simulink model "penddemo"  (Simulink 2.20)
settings: Solver=ode45  StartTime=0  StopTime=10000  MaxStep=0.02  RelTol=1e-3  AbsTol=1e-6

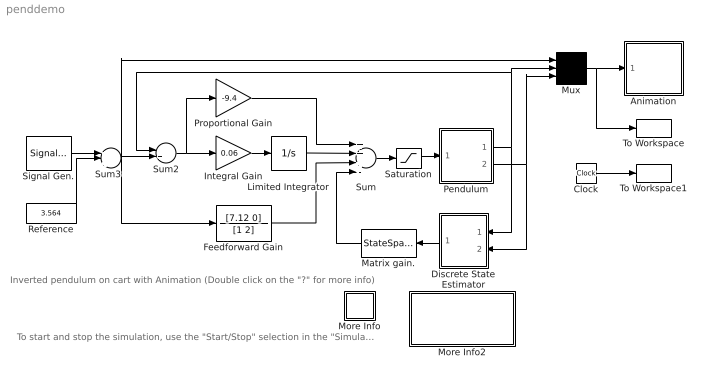
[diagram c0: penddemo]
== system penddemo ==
  note: Inverted pendulum on cart with Animation (Double click on the "?" for more info)
  note: To start and stop the simulation, use the "Start/Stop" selection in the "Simulation" pull-down menu
  Animation : Subsystem  mask(Pendulum plot){}
      mask help: Pendulum plot
      mask init:
      | RefBlock=&1;
  Clock : Clock
  Discrete State Estimator : Subsystem  Orientation=left  mask(Pendulum Discrete state estimator){}
      mask help: Pendulum discrete state estimator
      mask init:
      | Ts = @1;
  Feedforward Gain : TransferFcn  Numerator=[7.12 0]  Denominator=[1 2]
  Integral Gain : Gain  Gain=0.06
  Limited Integrator : Integrator  ExternalReset=none  InitialConditionSource=internal  InitialCondition=0  LimitOutput=on  UpperSaturationLimit=5  LowerSaturationLimit=-5  ShowSaturationPort=off  ShowStatePort=off  AbsoluteTolerance=auto
  Matrix gain. : StateSpace  Orientation=left  A=[]  B=[]  C=[]  D=K  X0=0  mask(Matrix gain){}
      mask help: Matrix Gain:
      mask init:
      | K = @1;
  More Info : Subsystem
  More Info2 : Subsystem
  Mux : Mux  Inputs=3
  Pendulum : Subsystem  mask(Inverted pendulum on cart){}
      mask help: Unmask and double-click to see dynamics
      mask init:
      | M=@1; m=@2; l=@3; g=@4;
  Proportional Gain : Gain  Gain=-9.4
  Reference : Constant  Value=3.564
  Saturation : Saturate  UpperLimit=10  LowerLimit=-10
  Signal Gen. : SignalGenerator  WaveForm=sine  Amplitude=5  Frequency=0.1  Units=Hertz
  Sum : Sum  Inputs=+++-
  Sum2 : Sum  Inputs=-+
  Sum3 : Sum  Inputs=+++
  To Workspace : ToWorkspace  VariableName=y  SampleTime=0.1
  To Workspace1 : ToWorkspace  VariableName=t  SampleTime=0.1
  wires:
  Sum2/1 -> Proportional Gain/1, Integral Gain/1
  Discrete State Estimator/1(X) -> Matrix gain./1
  Mux/1 -> To Workspace/1, Animation/1(in_1)
  Pendulum/2(Pendulum) -> Mux/3, Discrete State Estimator/2(Pendulum)
  Sum3/1 -> Mux/1, Feedforward Gain/1, Sum2/2
  Integral Gain/1 -> Limited Integrator/1
  Sum/1 -> Saturation/1
  Proportional Gain/1 -> Sum/1
  Feedforward Gain/1 -> Sum/3
  Reference/1 -> Sum3/2
  Signal Gen./1 -> Sum3/1
  Matrix gain./1 -> Sum/4
  Limited Integrator/1 -> Sum/2
  Pendulum/1(Cart) -> Sum2/1, Mux/2, Discrete State Estimator/1(Cart)
  Saturation/1 -> Pendulum/1(U)
  Clock/1 -> To Workspace1/1

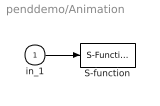
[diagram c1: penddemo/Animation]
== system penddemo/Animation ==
  in_1 : Inport  Port=1  PortWidth=-1  SampleTime=-1
  S-function : S-Function  FunctionName=pendan  Parameters=RefBlock  PortCounts=[]  SFunctionModules=''
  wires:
  in_1/1 -> S-function/1

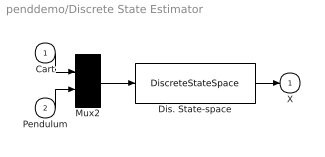
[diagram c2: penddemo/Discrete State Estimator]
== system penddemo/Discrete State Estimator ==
  Cart : Inport  Port=1  PortWidth=-1  SampleTime=-1
  Pendulum : Inport  Port=2  PortWidth=-1  SampleTime=-1
  Dis. State-space : DiscreteStateSpace  A=zeros(2)  B=-eye(2)/Ts  C=[0 0; 1 0; 0 0; 0 1]  D=[1 0; 1/Ts 0; 0 1; 0 1/Ts]  X0=0  SampleTime=Ts
  Mux2 : Mux  Inputs=2
  X : Outport  Port=1  InitialOutput=0
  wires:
  Pendulum/1 -> Mux2/2
  Dis. State-space/1 -> X/1
  Cart/1 -> Mux2/1
  Mux2/1 -> Dis. State-space/1

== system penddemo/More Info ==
  note: This system simulates a cart carrying an inverted pendulum and displays an animation.
  note: The animation is created using MATLAB's Handle Graphics. The animation block is just a masked S-function.
  note: For more information on what the S-function does, look at the functions pendan.m, pend0.m, and pendsets.m.

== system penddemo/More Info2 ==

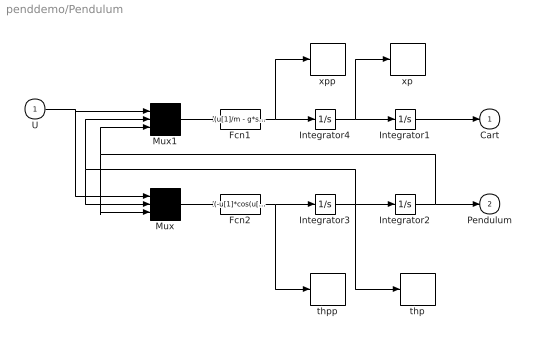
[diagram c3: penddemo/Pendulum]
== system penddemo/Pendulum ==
  U : Inport  Port=1  PortWidth=-1  SampleTime=-1
  Fcn1 : Fcn  Expr=(u[1]/m - g*sin(u[3])*cos(u[3]) + l*power(u[2],2)*sin(u[3]))/(M/m + power(sin(u[3]),2))
  Fcn2 : Fcn  Expr=(-u[1]*cos(u[3])/m + (M+m)*g*sin(u[3])/m - l*power(u[2],2)*sin(u[3])*cos(u[3]))/(l*(M/m + power(sin(u[3]),2)))
  Integrator{1..4} (4 alike) : Integrator  ExternalReset=none  InitialConditionSource=internal  InitialCondition=0  LimitOutput=off  UpperSaturationLimit=inf  LowerSaturationLimit=-inf  ShowSaturationPort=off  ShowStatePort=off  AbsoluteTolerance=auto
  Mux : Mux  Inputs=3
  Mux1 : Mux  Inputs=3
  thp : ToWorkspace  VariableName=thp  SampleTime=-1
  thpp : ToWorkspace  VariableName=thpp  SampleTime=-1
  xp : ToWorkspace  VariableName=xp  SampleTime=-1
  xpp : ToWorkspace  VariableName=xpp  SampleTime=-1
  Cart : Outport  Port=1  InitialOutput=0
  Pendulum : Outport  Port=2  InitialOutput=0
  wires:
  Integrator1/1 -> Cart/1
  Mux/1 -> Fcn2/1
  Mux1/1 -> Fcn1/1
  U/1 -> Mux1/1, Mux/1
  Integrator3/1 -> Integrator2/1, Mux1/2, Mux/2, thp/1
  Integrator2/1 -> Pendulum/1, Mux1/3, Mux/3
  Fcn2/1 -> Integrator3/1, thpp/1
  Fcn1/1 -> Integrator4/1, xpp/1
  Integrator4/1 -> Integrator1/1, xp/1
